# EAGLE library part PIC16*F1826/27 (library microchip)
18/20/28-Pin Flash Microcontrollers with nanoWatt XLP Technology Source: www.microchip.com PIC16F1827.pdf
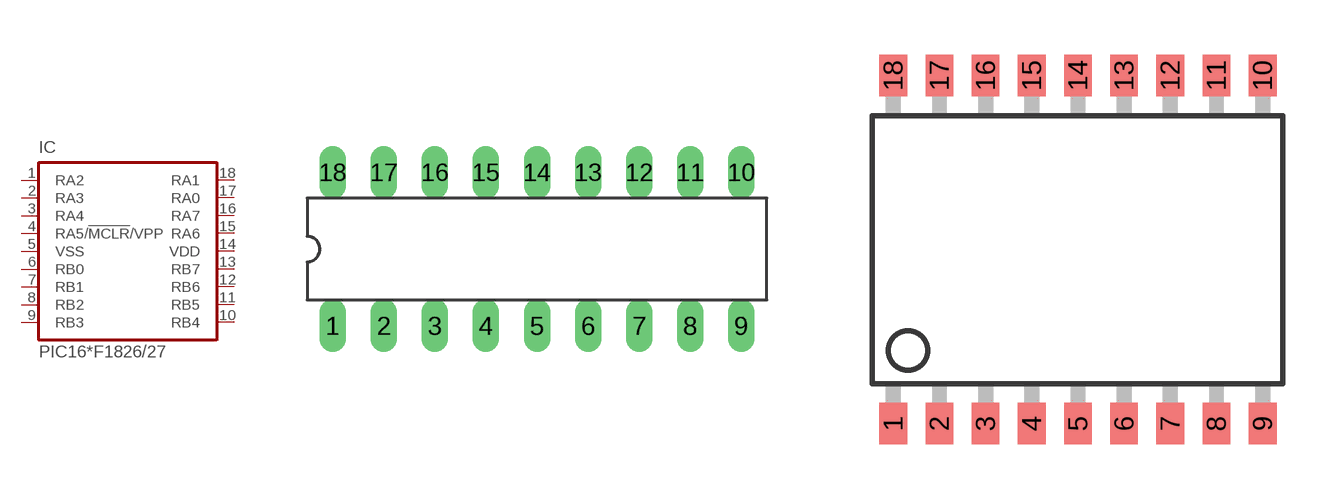
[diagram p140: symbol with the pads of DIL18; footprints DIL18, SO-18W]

Designator prefix IC

## PIC16F1826/27P, PIC16LF1826/27P  [DIL18]
1  RA2
2  RA3
3  RA4
4  RA5/!MCLR!/VPP
5  VSS  pwr
6  RB0
7  RB1
8  RB2
9  RB3
10  RB4
11  RB5
12  RB6
13  RB7
14  VDD  pwr
15  RA6
16  RA7
17  RA0
18  RA1

## PIC16F1826/27SO, PIC16LF1826/27SO  [SO-18W]
Pads as for DIL18

## PIC16F1826/27SS, PIC16LF1826/27SS  [SSOP20]
1  RA2
2  RA3
3  RA4
4  RA5/!MCLR!/VPP
5  VSS  pwr
6  VSS  pwr
7  RB0
8  RB1
9  RB2
10  RB3
11  RB4
12  RB5
13  RB6
14  RB7
15  VDD  pwr
16  VDD  pwr
17  RA6
18  RA7
19  RA0
20  RA1

## PIC16F1826/27ML, PIC16LF1826/27ML  [QFN28]
1  RA5/!MCLR!/VPP
3  VSS  pwr
5  VSS  pwr
7  RB0
8  RB1
9  RB2
10  RB3
12  RB4
13  RB5
15  RB6
16  RB7
17  VDD  pwr
19  VDD  pwr
20  RA6
21  RA7
23  RA0
24  RA1
26  RA2
27  RA3
28  RA4

## Footprint DIL18 (pad centres in mm)
Dual In Line package type P
drill 0.813 long: 1 -10.16,-3.81; 2 -7.62,-3.81; 3 -5.08,-3.81; 4 -2.54,-3.81; 5 0,-3.81; 6 2.54,-3.81; 7 5.08,-3.81; 8 7.62,-3.81; 9 10.16,-3.81; 10 10.16,3.81; 11 7.62,3.81; 12 5.08,3.81; 13 2.54,3.81; 14 0,3.81; 15 -2.54,3.81; 16 -5.08,3.81; 17 -7.62,3.81; 18 -10.16,3.81

## Footprint SO-18W (pad centres in mm)
Small Outline Wide Plastic Gull Wing 300-mil body, package type SO
smd 0.762 x 1.143: 1 -5.08,-4.788; 2 -3.81,-4.788; 3 -2.54,-4.788; 4 -1.27,-4.788; 5 0,-4.788; 6 1.27,-4.788; 7 2.54,-4.788; 8 3.81,-4.788; 9 5.08,-4.788; 10 5.08,4.788; 11 3.81,4.788; 12 2.54,4.788; 13 1.27,4.788; 14 0,4.788; 15 -1.27,4.788; 16 -2.54,4.788; 17 -3.81,4.788; 18 -5.08,4.788

## Footprint SSOP20 (pad centres in mm)
Shrink Small Outline Package package type SS
smd 0.4 x 1.5: 1 -2.925,-3.625; 2 -2.275,-3.625; 3 -1.625,-3.625; 4 -0.975,-3.625; 5 -0.325,-3.625; 6 0.325,-3.625; 7 0.975,-3.625; 8 1.625,-3.625; 9 2.275,-3.625; 10 2.925,-3.625; 11 2.925,3.625; 12 2.275,3.625; 13 1.625,3.625; 14 0.975,3.625; 15 0.325,3.625; 16 -0.325,3.625; 17 -0.975,3.625; 18 -1.625,3.625; 19 -2.275,3.625; 20 -2.925,3.625

## Footprint QFN28 (pad centres in mm)
28-Lead Plastic Quad Flat No Lead Package (ML) 6x6 mm Body, Punch Singulated (QFN) Source: ww1.microchip.com/downloads/en/DeviceDoc/39605c.pdf
smd 0.8 x 0.4: 1 -2.65,1.95; 2 -2.65,1.3; 3 -2.65,0.65; 4 -2.65,0; 5 -2.65,-0.65; 6 -2.65,-1.3; 7 -2.65,-1.95; 15 2.65,-1.95; 16 2.65,-1.3; 17 2.65,-0.65; 18 2.65,0; 19 2.65,0.65; 20 2.65,1.3; 21 2.65,1.95
smd 0.4 x 0.8: 8 -1.95,-2.65; 9 -1.3,-2.65; 10 -0.65,-2.65; 11 0,-2.65; 12 0.65,-2.65; 13 1.3,-2.65; 14 1.95,-2.65; 22 1.95,2.65; 23 1.3,2.65; 24 0.65,2.65; 25 0,2.65; 26 -0.65,2.65; 27 -1.3,2.65; 28 -1.95,2.65
smd 3.55 x 3.55: M 0,0
smd 0.17 x 0.4 rotated 45: R1 -2.525,2.525
smd 0.17 x 0.4 rotated 135: R2 -2.525,-2.525
smd 0.17 x 0.4 rotated 225: R3 2.525,-2.525
smd 0.17 x 0.4 rotated 315: R4 2.5,2.5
